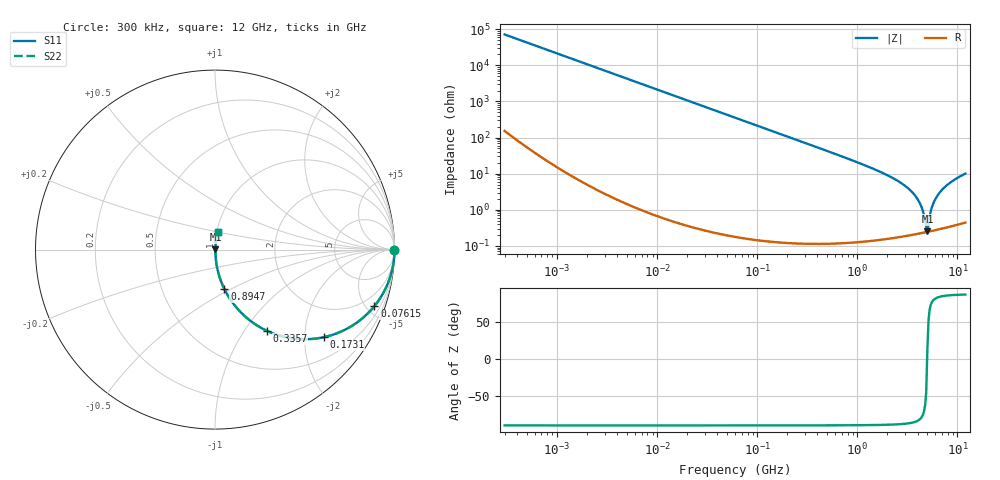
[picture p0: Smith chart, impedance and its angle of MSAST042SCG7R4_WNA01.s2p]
! MSAST042SCG7R4_WNA01  S-PARAMETER MODEL  ( General Type )
! Model Generated by TAIYO YUDEN Corporation (http://www.ty-top.com)
! Version 1.0
! TAIYO YUDEN Control No. 150820
! Copyright(c) 2015 TAIYO YUDEN CO.,LTD. All Rights Reserved.
! Product Description (link to TY-COMPAS)
! https://ds.yuden.co.jp/TYCOMPAS/or/detail?pn=MSAST042SCG7R4BWNA01&u=M
! Products Name : Multilayer Ceramic Capacitors
! Characteristics :
!  Capacitance : 7.4 pF , Rated Voltage : 25V , TCC : CG / C0G
!  Case Size : 0.4 x 0.2 / 0.016 x 0.008 [mm/inch] , Thickness : 0.2 / 0.008 [mm/inch]
!  (Conditions: Temperature = 25 degC , DC Bias Current/Voltage = 0A / 0V)
! External Node Assignments :
!  1  o---| |---o  2
! GND o---------o GND
! Frequency Range : 0.3MHz  -  12000MHz  [ 401 STEP ]
# MHz S RI R 50
! Freq[MHz].  S11 Real  S11 Imag  S21 Real  S21 Imag  S12 Real  S12 Imag  S22 Real  S22 Imag
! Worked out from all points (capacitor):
!   401 points, 300 kHz to 12 GHz, reference 50 ohm
!   read as one part in series: C = 7.4 pF near 316.3 kHz
!   lowest |Z| = 251 mohm at 5.006 GHz (marker M1)
!   series resonance near 4.981 GHz, so ESL is about 140 pH
!   S11 on the Smith chart (normalised r, x): 300 kHz: open; 76.15 MHz: 1.00, -5.65; 173.1 MHz: 1.00, -2.48; 335.7 MHz: 1.00, -1.28; 894.7 MHz: 1.00, -0.47; 12 GHz: 1.01, +0.20
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0.3  1 -0.0014  4.92e-06 0.0014  4.92e-06 0.0014  1 -0.0014
1.769972  0.9999 -0.00823  7.18e-05 0.00823  7.18e-05 0.00823  0.9999 -0.00823
10.44266  0.9976 -0.0485  0.00237 0.0485  0.00237 0.0485  0.9976 -0.0485
27.10171  0.9843 -0.1241  0.0157 0.1241  0.0157 0.1241  0.9843 -0.1241
60  0.9276 -0.2589  0.0724 0.2589  0.0724 0.2589  0.9276 -0.2589
76.15486  0.8884 -0.3147  0.1116 0.3147  0.1116 0.3147  0.8884 -0.3147
173.124  0.606 -0.4881  0.394 0.4881  0.394 0.4881  0.606 -0.4881
335.7268  0.2894 -0.4526  0.7106 0.4526  0.7106 0.4526  0.2894 -0.4526
353.9943  0.2679 -0.4419  0.7321 0.4419  0.7321 0.4419  0.2679 -0.4419
894.6982  0.0524 -0.2202  0.9476 0.2202  0.9476 0.2202  0.0524 -0.2202
2088.533  0.00874 -0.0842  0.9913 0.0842  0.9913 0.0842  0.00874 -0.0842
2947.191  0.0041 -0.0475  0.9959 0.0475  0.9959 0.0475  0.0041 -0.0475
3740.715  0.00272 -0.0254  0.9973 0.0254  0.9973 0.0254  0.00272 -0.0254
4270.516  0.00242 -0.0138  0.9976 0.0138  0.9976 0.0138  0.00242 -0.0138
4502.883  0.00238 -0.00919  0.9976 0.00919  0.9976 0.00919  0.00238 -0.00919
4747.894  0.00238 -0.00465  0.9976 0.00465  0.9976 0.00465  0.00238 -0.00465
5006.236  0.00244 0.000566  0.9976 -0.000566  0.9976 -0.000566  0.00244 0.000566
5140.631  0.00249 0.00327  0.9975 -0.00327  0.9975 -0.00327  0.00249 0.00327
5715.274  0.00284 0.0143  0.9972 -0.0143  0.9972 -0.0143  0.00284 0.0143
6699.894  0.00384 0.0304  0.9962 -0.0304  0.9962 -0.0304  0.00384 0.0304
8503.825  0.00661 0.0563  0.9934 -0.0563  0.9934 -0.0563  0.00661 0.0563
12000  0.0142 0.0983  0.9858 -0.0983  0.9858 -0.0983  0.0142 0.0983
